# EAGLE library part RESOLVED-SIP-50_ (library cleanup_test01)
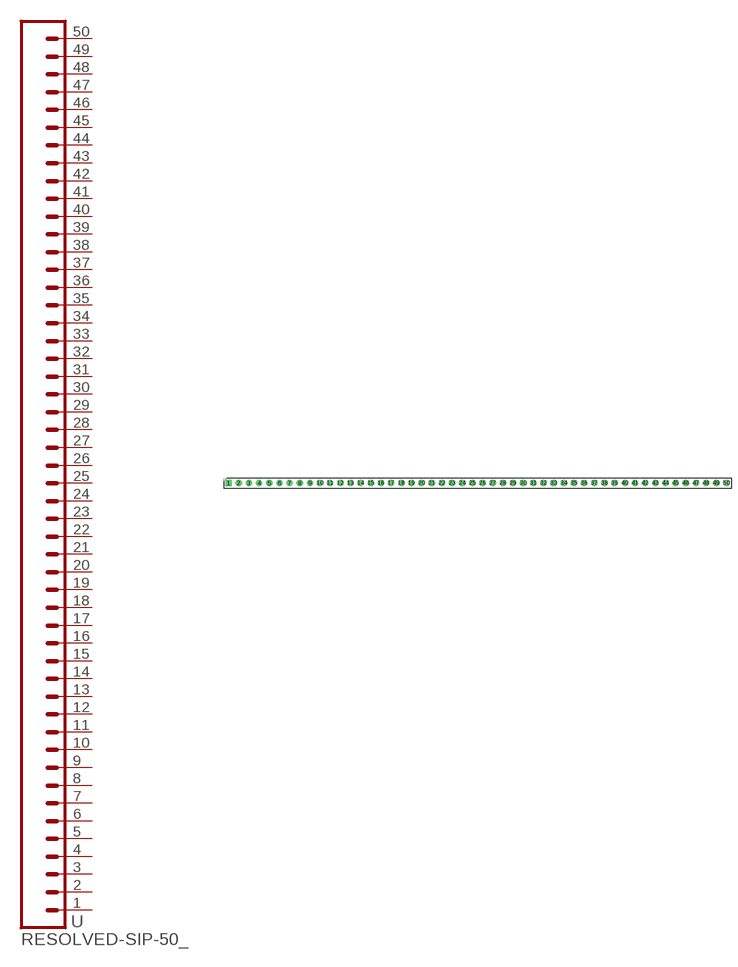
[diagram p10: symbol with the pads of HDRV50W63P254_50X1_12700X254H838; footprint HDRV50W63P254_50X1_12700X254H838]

Designator prefix -

## RESOLVED-SIP-50_BREAKABLE-2.54-SPACE-VERTICAL  [HDRV50W63P254_50X1_12700X254H838]
1  1  pas
2  2  pas
3  3  pas
4  4  pas
5  5  pas
6  6  pas
7  7  pas
8  8  pas
9  9  pas
10  10  pas
11  11  pas
12  12  pas
13  13  pas
14  14  pas
15  15  pas
16  16  pas
17  17  pas
18  18  pas
19  19  pas
20  20  pas
21  21  pas
22  22  pas
23  23  pas
24  24  pas
25  25  pas
26  26  pas
27  27  pas
28  28  pas
29  29  pas
30  30  pas
31  31  pas
32  32  pas
33  33  pas
34  34  pas
35  35  pas
36  36  pas
37  37  pas
38  38  pas
39  39  pas
40  40  pas
41  41  pas
42  42  pas
43  43  pas
44  44  pas
45  45  pas
46  46  pas
47  47  pas
48  48  pas
49  49  pas
50  50  pas

## Footprint HDRV50W63P254_50X1_12700X254H838 (pad centres in mm)
drill 1.1 pad 1.65 square: 1 0,0
drill 1.1 pad 1.65: 2 2.54,0; 3 5.08,0; 4 7.62,0; 5 10.16,0; 6 12.7,0; 7 15.24,0; 8 17.78,0; 9 20.32,0; 10 22.86,0; 11 25.4,0; 12 27.94,0; 13 30.48,0; 14 33.02,0; 15 35.56,0; 16 38.1,0; 17 40.64,0; 18 43.18,0; 19 45.72,0; 20 48.26,0; 21 50.8,0; 22 53.34,0; 23 55.88,0; 24 58.42,0; 25 60.96,0; 26 63.5,0; 27 66.04,0; 28 68.58,0; 29 71.12,0; 30 73.66,0; 31 76.2,0; 32 78.74,0; 33 81.28,0; 34 83.82,0; 35 86.36,0; 36 88.9,0; 37 91.44,0; 38 93.98,0; 39 96.52,0; 40 99.06,0; 41 101.6,0; 42 104.14,0; 43 106.68,0; 44 109.22,0; 45 111.76,0; 46 114.3,0; 47 116.84,0; 48 119.38,0; 49 121.92,0; 50 124.46,0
